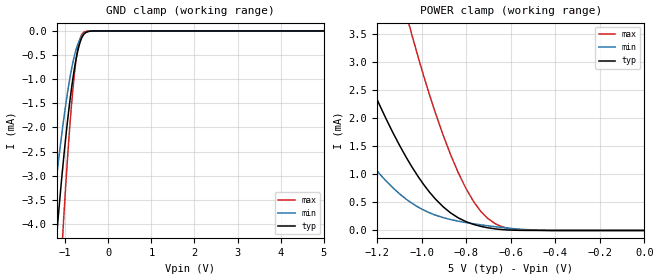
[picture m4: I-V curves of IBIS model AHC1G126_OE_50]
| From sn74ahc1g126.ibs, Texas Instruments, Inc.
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[Model]   AHC1G126_OE_50
Model_type  Input
Vinl=1.65
Vinh=3.85
| variable   typ   min   max
C_comp   2.66pF   2.26pF   2.87pF
[Temperature Range]   40   100   -40
| Ambient temperature   25   85   -40
[Voltage range]   5   4.5   5.5
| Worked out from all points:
|   GND clamp passes 1 mA (typ) near -0.82 V on its own axis
|   POWER clamp passes 1 mA (typ) near -1.02 V on its own axis
[GND Clamp]
| AHC1G126_OE_50
|   Voltage   I(typ)   I(min)   I(max)
-5V       -82.2mA    -53.18mA   -120.1mA
-1.345V   -5.939mA   -4.23mA    -9.455mA
-1.325V   -5.698mA   -4.059mA   -9.052mA
-1.18V    -4.064mA   -2.884mA   -6.306mA
-1.08V    -3.056mA   -2.15mA    -4.612mA
-1.045V   -2.728mA   -1.909mA   -4.063mA
-900mV    -1.524mA   -1.032mA   -2.071mA
-825mV    -1.015mA   -673.6uA   -1.254mA
-760mV    -650.5uA   -429.5uA   -694.5uA
-660mV    -253.8uA   -181.4uA   -175.8uA
-540mV    -43.74uA   -45.9uA    -14.62uA
5V        202.2pA    7.882uA    5.191pA
[POWER Clamp]
| AHC1G126_OE_50
|   Voltage   I(typ)   I(min)   I(max)
-5V       84.23mA    53.81mA    136.8mA
-1.595V   6.677mA    3.573mA    14.16mA
-1.34V    3.677mA    1.806mA    8.607mA
-1.19V    2.243mA    1.013mA    5.808mA
-1.07V    1.306mA    558.7uA    3.866mA
-1.045V   1.14mA     487.9uA    3.498mA
-940mV    566.9uA    276.1uA    2.112mA
-835mV    223.3uA    164.8uA    1.022mA
-765mV    105.5uA    117.7uA    503.4uA
-705mV    49.45uA    84.73uA    220uA
-580mV    3.937uA    29.62uA    18.37uA
-84.45fV  202.2pA    739.6pA    6.479pA
